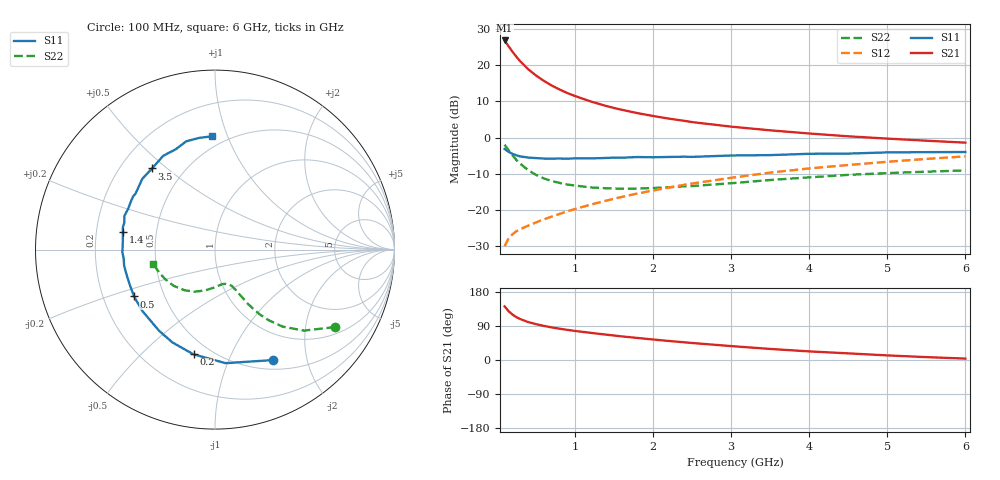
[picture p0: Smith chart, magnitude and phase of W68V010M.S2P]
! SIEMENS Small Signal Semiconductors
! BFR193W
! Si NPN RF Bipolar Junction Transistor in SOT323
! VCE = 8 V  IC = 10 mA
! Common Emitter S-Parameters:  September  1992
# GHz  S  MA  R  50
!  f  S11  S21  S12  S22
! GHz  MAG  ANG  MAG  ANG  MAG  ANG  MAG  ANG
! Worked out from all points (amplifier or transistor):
!   28 points, 100 MHz to 6 GHz, reference 50 ohm
!   highest |S21| = 26.7 dB at 100 MHz (marker M1)
!   |S21| within 3 dB of that: start of sweep to 197.4 MHz
!   unconditionally stable (mu >= 1): 1.039 GHz to 2.618 GHz
!   at 300 MHz: K = 0.55, MSG = 23.1 dB, |S12| = -25.3 dB
!   at 1.5 GHz: K = 1.04, MAG = 11.2 dB, |S12| = -16.9 dB
!   at 6 GHz: K = 0.89, MSG = 1.9 dB, |S12| = -5.2 dB
!   lowest NFmin = 1.30 dB at 450 MHz
!   S11 on the Smith chart (normalised r, x): 100 MHz: 0.62, -1.47; 200 MHz: 0.40, -0.73; 500 MHz: 0.34, -0.24; 1.4 GHz: 0.32, +0.09; 3.5 GHz: 0.33, +0.45; 6 GHz: 0.42, +0.88
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0.1  0.6947 -62.4  21.7 141.6  0.0319 62.3  0.7965 -32.8
0.15  0.6354 -84.7  18.11 129.0  0.0406 55.5  0.6705 -42.3
0.2  0.5956 -101.6  15.23 119.9  0.0464 51.5  0.5714 -48.7
0.25  0.5691 -114.6  12.96 113.2  0.0511 49.8  0.4918 -52.9
0.3  0.5494 -124.5  11.23 108.0  0.0546 49.2  0.4364 -55.5
0.4  0.5299 -139.9  8.763 100.2  0.0611 50.0  0.356 -58.7
0.5  0.521 -149.9  7.166 94.7  0.0676 51.6  0.3066 -60.3
0.6  0.5134 -158.2  6.052 90.1  0.0746 53.5  0.2739 -61.9
0.7  0.5122 -164.6  5.213 86.1  0.0812 55.2  0.2524 -62.8
0.8  0.5141 -170.0  4.604 82.7  0.0883 56.8  0.2375 -64.1
0.9  0.5111 -174.4  4.107 79.6  0.096 58.2  0.2254 -64.9
1  0.5164 -178.4  3.733 76.7  0.1035 59.3  0.218 -66.1
1.2  0.5156 174.6  3.141 71.7  0.119 61.0  0.2054 -69.4
1.4  0.523 169.2  2.719 66.9  0.1351 62.0  0.2001 -72.6
1.8  0.5385 159.5  2.169 58.2  0.1694 63.0  0.1982 -80.3
2.2  0.5397 150.4  1.823 50.3  0.2045 62.6  0.2063 -87.8
2.5  0.5412 144.9  1.631 44.9  0.2321 61.7  0.2148 -93.6
3  0.5654 135.8  1.412 36.7  0.2788 59.5  0.2344 -103.8
3.5  0.5723 127.8  1.256 29.2  0.3288 56.2  0.26 -115.6
4.5  0.6006 111.2  1.039 17.5  0.4182 48.3  0.3061 -138.7
5.5  0.6287 98.1  0.904 7.6  0.5071 40.0  0.3384 -159.3
6  0.6313 91.5  0.85 3.7  0.5496 35.2  0.3524 -166.5
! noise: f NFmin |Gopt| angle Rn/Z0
0.45  1.3  0.22  143  0.11
0.9  1.3  0.34  160  0.11
1.8  2.05  0.54  -153  0.14
